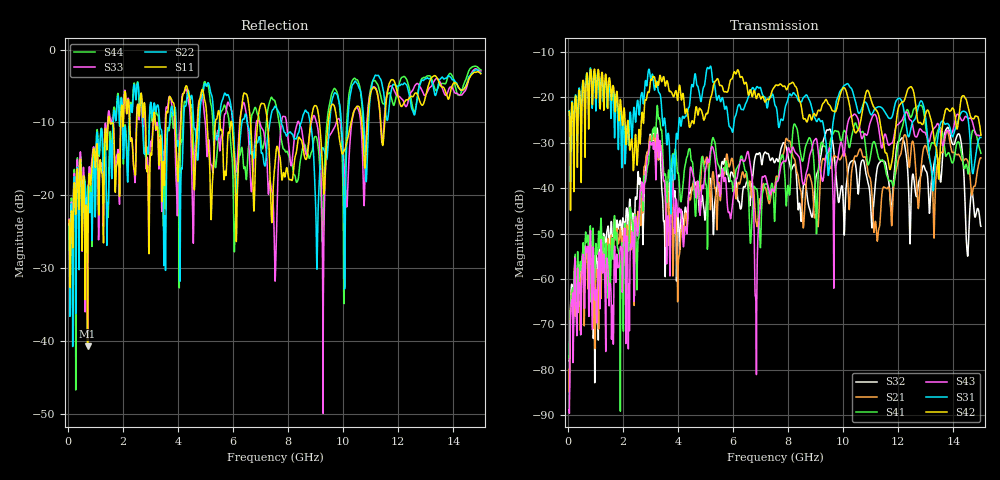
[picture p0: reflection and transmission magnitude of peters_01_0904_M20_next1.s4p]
# MHZ S RI R 50.00
! FREQ  S11  S12  S13  S14
!  S21  S22  S23  S24
!  S31  S32  S33  S34
!  S41  S42  S43  S44
!  REAL  IMAG  REAL  IMAG  REAL  IMAG  REAL  IMAG
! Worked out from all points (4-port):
!   1496 points, 50 MHz to 15 GHz, reference 50 ohm
!   strongest paths, dB at 50 MHz, 3.79 GHz, 7.53 GHz, 11.27 GHz, 15 GHz:
!     S42: -23.1, -19.2, -17.4, -23.5, -28.3
!     S31: -22.9, -35.6, -21.8, -22.1, -28.8
!     S43: -88.8, -39.3, -40.0, -26.0, -28.1
!     S41: -77.4, -33.0, -44.7, -33.0, -32.3
!     S21: -79.9, -45.4, -38.9, -50.0, -33.3
!     S32: -78.0, -36.2, -34.2, -34.8, -48.4
!   lowest |S11| = -40.7 dB at 720 MHz (marker M1), VSWR 1.02, Z = 49.7 + j0.871 ohm
!   |S11| at or under -10 dB: start of sweep to 1.464 GHz; 7.252 GHz to 8.821 GHz (1.569 GHz wide, 19.5 % of centre); 9.788 GHz to 10.29 GHz (500 MHz wide, 4.98 % of centre)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
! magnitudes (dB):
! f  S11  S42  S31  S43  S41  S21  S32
! 50 MHz  -23.4  -23.1  -22.9  -88.8  -77.4  -79.9  -78.0
! 720 MHz  -40.7  -16.0  -16.0  -53.9  -51.1  -59.6  -54.6
! 3.19 GHz  -10.4  -17.1  -17.0  -35.9  -28.7  -34.0  -30.5
! 6.54 GHz  -6.8  -18.9  -20.2  -31.9  -38.8  -39.7  -39.0
! 6.84 GHz  -13.1  -20.2  -17.9  -69.4  -40.1  -47.6  -32.5
! 8.03 GHz  -17.8  -17.2  -19.5  -31.2  -40.6  -29.6  -33.9
! 15 GHz  -3.3  -28.3  -28.8  -28.1  -32.3  -33.3  -48.4
